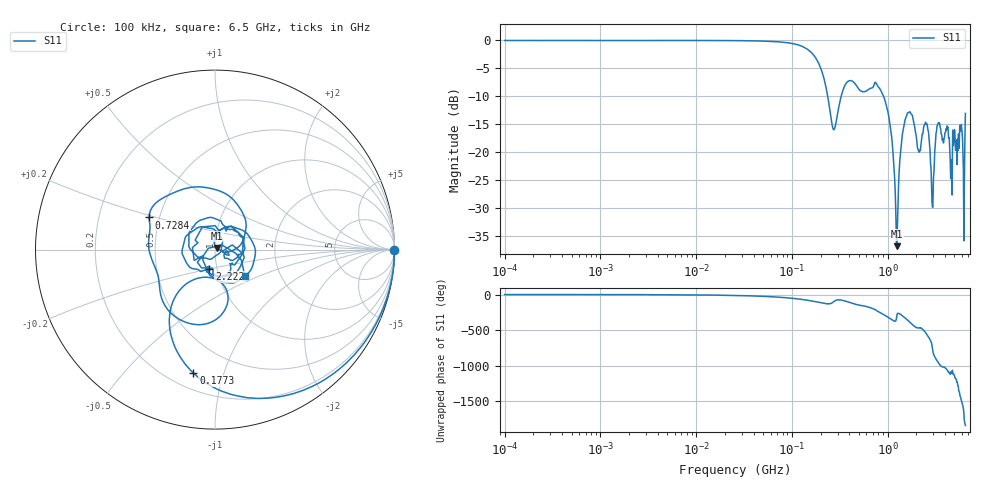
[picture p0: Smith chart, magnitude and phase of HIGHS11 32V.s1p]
!Keysight Technologies,E5080B,MY59100498,A.17.05.10
!Date: Wednesday, August 30, 2023 19:25:44
!Correction: S11(C  1-Port  )
!S1P File: Measurement: S11:Log Frequency Sweep
# Hz S  dB  R 50
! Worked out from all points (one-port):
!   1601 points, 100 kHz to 6.5 GHz, reference 50 ohm
!   lowest |S11| = -36.9 dB at 1.242 GHz (marker M1), VSWR 1.03, Z = 51.2 + j0.856 ohm
!   |S11| at or under -10 dB: 236.9 MHz to 327.8 MHz (90.87 MHz wide, 32.2 % of centre); 908 MHz to end of sweep
!   S11 on the Smith chart (normalised r, x): 100 kHz: open; 177.3 MHz: 0.30, -0.80; 728.4 MHz: 0.44, +0.19; 2.222 GHz: 0.92, -0.20; 6.5 GHz: 1.33, -0.41
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100000  -0.00 -0.1
399589.6  -0.00 -0.2
1596718  -0.00 -0.8
6380321  -0.00 -3.1
2.54951e7  -0.03 -12.8
5.894314e7  -0.16 -29.9
1.018758e8  -0.55 -53.3
1.401013e8  -1.40 -76.2
1.773032e8  -3.12 -99.9
2.182522e8  -7.05 -124.7
2.724062e8  -15.97 -103.3
3.28424e8  -9.95 -78.1
4.070849e8  -7.20 -114.0
7.283883e8  -7.78 154.0
8.541784e8  -9.04 100.3
1.022724e9  -13.33 36.3
1.241608e9  -36.89 35.8
1.416243e9  -17.37 65.5
1.626669e9  -12.94 -2.2
1.829938e9  -13.78 -65.3
2.221582e9  -19.00 -106.7
2.551666e9  -15.05 164.6
2.930793e9  -29.43 -26.0
3.389649e9  -14.78 121.4
4.201505e9  -15.50 17.7
4.661503e9  -21.43 -21.3
5.317155e9  -22.25 -153.0
6.5e9  -13.08 -41.5
